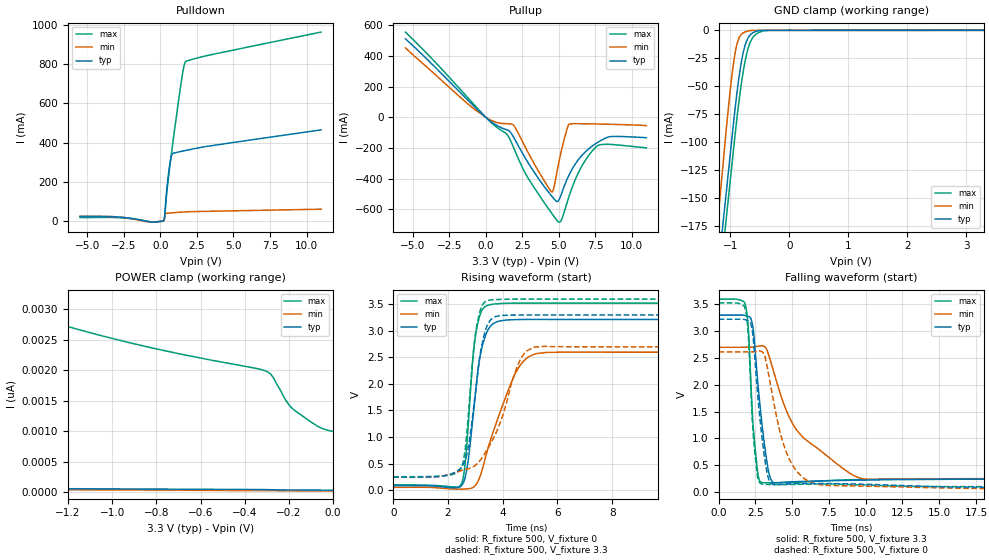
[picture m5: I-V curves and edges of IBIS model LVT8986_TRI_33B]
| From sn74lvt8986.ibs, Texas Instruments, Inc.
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[Model]   LVT8986_TRI_33B
Model_type  3-state
Enable   Active-Low
Vref =   0
Rref =   500
Cref =   50p
Vmeas =   1.5
| variable   typ   min   max
C_comp   6.45pF   5.13pF   10.40pF
| C_pullup   7.55pF   0.34pF   21.55pF
| C_pulldown   8.23pF   1.62pF   16.10pF
| C_tri-state   6.45pF   5.13pF   10.40pF
[Temperature Range]   40   -40   100
| Ambient temperature   25   -40   85
[Voltage range]   3.3   2.7   3.6
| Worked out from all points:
|   slope of the pulldown table from 0 to 0.495 V, typ, clamps not added: 2.41 ohm
|   slope of the pullup table from 0 to 0.495 V, typ, clamps not added: 13.2 ohm
|   GND clamp passes 1 mA (typ) near -0.57 V on its own axis
|   rising waveform, R_fixture 500, V_fixture 0: 20-80 % time 424ps typ, 1.02ns min, 309ps max; typ from 0.084 V to 3.22 V
|   falling waveform, R_fixture 500, V_fixture 3.3: 20-80 % time 659ps typ, 3.32ns min, 401ps max; typ from 3.3 V to 0.242 V
|   rising waveform, R_fixture 500, V_fixture 3.3: 20-80 % time 464ps typ, 1.05ns min, 341ps max; typ from 0.243 V to 3.3 V
|   falling waveform, R_fixture 500, V_fixture 0: 20-80 % time 650ps typ, 1.44ns min, 407ps max; typ from 3.22 V to 0.085 V
[GND Clamp]
| LVT8986_TRI_33B
|   Voltage   I(typ)   I(min)   I(max)
-5.5V     -3.218A    -3.568A    -3.44A
-1.24V    -230.7mA   -185.6mA   -254.6mA
-1.075V   -147.4mA   -91.35mA   -170.9mA
-975mV    -97.12mA   -40.67mA   -120.7mA
-925mV    -72.35mA   -21.76mA   -95.72mA
-875mV    -50.21mA   -9.741mA   -72.33mA
-800mV    -24.3mA    -2.921mA   -42.48mA
-725mV    -9.521mA   -995.2uA   -21.21mA
-650mV    -3.38mA    -201.3uA   -9.148mA
-575mV    -1.037mA   -9.75uA    -3.834mA
-325mV    -396nA     -603.8pA   -16.32uA
3.3V      31.85pA    30.31pA    905.7pA
[POWER Clamp]
| LVT8986_TRI_33B
|   Voltage   I(typ)   I(min)   I(max)
-5.5V     128.1pA    102.9pA    27.52nA
-1.655V   63.6pA     45.87pA    3.266nA
-1.54V    61.75pA    44.24pA    3.112nA
-1.305V   57.98pA    40.95pA    2.83nA
-930mV    52.01pA    35.75pA    2.46nA
-305mV    41.22pA    23.79pA    1.989nA
-290mV    40.2pA     23.62pA    1.959nA
-275mV    39.05pA    23.46pA    1.902nA
-215mV    36.17pA    22.82pA    1.511nA
-180mV    35.16pA    22.44pA    1.359nA
-70mV     32.92pA    21.26pA    1.081nA
-95.1fV   31.84pA    20.51pA    997.6pA
[Pulldown]
| LVT8986_TRI_33B
|   Voltage   I(typ)   I(min)   I(max)
-5.5V     24.53mA    25.46mA    18.65mA
-2.815V   21.54mA    21.34mA    18.15mA
-685mV    -3.267mA   -4.141mA   -2.466mA
235mV     4.474mA    3.982mA    4.103mA
300mV     36.31mA    23.25mA    27.35mA
415mV     145.2mA    40.54mA    130.3mA
535mV     230.4mA    41.48mA    212.5mA
760mV     335.2mA    42.87mA    347.5mA
1.48V     356.3mA    46.85mA    734.4mA
1.63V     358.7mA    47.54mA    795mA
1.745V    360.6mA    48.02mA    813.3mA
11V       465mA      61.55mA    962.3mA
[Pullup]
| LVT8986_TRI_33B
|   Voltage   I(typ)   I(min)   I(max)
-5.5V     511mA      451.9mA    554.3mA
-640mV    56.77mA    42.3mA     65.8mA
1.435V    -81.32mA   -41.71mA   -109.8mA
1.89V     -126.4mA   -50.79mA   -193.3mA
2.79V     -278.4mA   -209.4mA   -378.3mA
4.5V      -510.8mA   -485.2mA   -622.3mA
4.655V    -528.8mA   -463.3mA   -643.1mA
5V        -540.3mA   -297.1mA   -682.2mA
5.685V    -379.5mA   -46.9mA    -520.5mA
6.535V    -253.8mA   -42.29mA   -325.5mA
7.595V    -167.5mA   -43.81mA   -189.3mA
11V       -133.6mA   -54.14mA   -199.7mA
[Ramp]
| LVT8986_TRI_33B
| variable   typ   min   max
dV/dt_r   1.90/4.33E-10   1.55/1.04E-09   2.08/3.18E-10
dV/dt_f   1.88/6.86E-10   1.50/3.34E-09   2.06/4.26E-10
R_load = 500
[Rising Waveform]
| LVT8986_TRI_33B
R_fixture =   500
C_fixture =   0
L_fixture =   0
V_fixture =   0
V_fixture_min = 0
V_fixture_max = 0
|   Time   V(typ)   V(min)   V(max)
0s        84.12mV    51.14mV    97.75mV
2.485ns   80.32mV    16.96mV    116.2mV
2.715ns   481.4mV    24.01mV    1.059V
2.895ns   1.291V     45.07mV    2.403V
3.015ns   1.886V     97.82mV    2.954V
3.19ns    2.573V     287.8mV    3.331V
3.49ns    3.047V     837.1mV    3.49V
4.48ns    3.214V     2.219V     3.524V
5.285ns   3.217V     2.577V     3.525V
24.99ns   3.217V     2.599V     3.525V
[Falling Waveform]
| LVT8986_TRI_33B
R_fixture =   500
C_fixture =   0
L_fixture =   0
V_fixture =   3.3
V_fixture_min = 2.7
V_fixture_max = 3.6
|   Time   V(typ)   V(min)   V(max)
0s        3.3V       2.7V       3.6V
1.84ns    3.29V      2.701V     3.468V
2.035ns   3.275V     2.702V     2.981V
2.32ns    3.093V     2.703V     1.344V
2.845ns   1.536V     2.728V     183.5mV
3.37ns    420.4mV    2.584V     172.6mV
3.72ns    172.9mV    2.268V     173.1mV
5.355ns   193mV      1.141V     181.9mV
9.4ns     220.1mV    279.2mV    229.4mV
24.99ns   241.7mV    240.7mV    250.4mV
[Rising Waveform]
| LVT8986_TRI_33B
R_fixture =   500
C_fixture =   0
L_fixture =   0
V_fixture =   3.3
V_fixture_min = 2.7
V_fixture_max = 3.6
|   Time   V(typ)   V(min)   V(max)
0s        243.4mV    240.9mV    251.8mV
2.47ns    414.5mV    365.3mV    409.2mV
2.64ns    584.3mV    390mV      832.2mV
2.9ns     1.403V     432.3mV    2.456V
3.035ns   1.981V     481.8mV    3.057V
3.23ns    2.722V     601.4mV    3.464V
3.48ns    3.152V     806.9mV    3.578V
4.64ns    3.299V     2.458V     3.601V
5.195ns   3.3V       2.697V     3.601V
24.99ns   3.3V       2.7V       3.6V
[Falling Waveform]
| LVT8986_TRI_33B
R_fixture =   500
C_fixture =   0
L_fixture =   0
V_fixture =   0
V_fixture_min = 0
V_fixture_max = 0
|   Time   V(typ)   V(min)   V(max)
0s        3.223V     2.613V     3.529V
1.835ns   3.213V     2.614V     3.389V
2.03ns    3.192V     2.614V     2.879V
2.425ns   2.644V     2.618V     841.3mV
2.66ns    1.809V     2.628V     269.6mV
2.905ns   1.124V     2.624V     150.2mV
3.535ns   164.8mV    1.992V     139.6mV
4.69ns    148.4mV    686.1mV    139mV
6.315ns   157.5mV    175.1mV    147.5mV
24.99ns   84.67mV    52.18mV    98.16mV
